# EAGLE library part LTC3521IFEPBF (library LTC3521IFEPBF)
DC/DC Converters Source: Datasheet
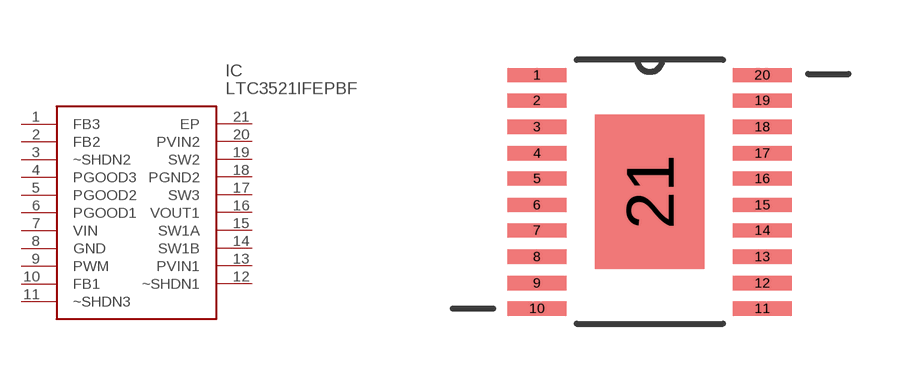
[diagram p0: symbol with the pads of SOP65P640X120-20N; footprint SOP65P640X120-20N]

Designator prefix IC

## LTC3521IFEPBF (Arrow_Part_Number: LTC3521IFEPBF; Description: DC/DC Converters; Height: mm; Manufacturer_Name: Linear Technology; Manufacturer_Part_Number: LTC3521IFEPBF)  [SOP65P640X120-20N]
1  FB3
2  FB2
3  ~SHDN2
4  PGOOD3
5  PGOOD2
6  PGOOD1
7  VIN
8  GND
9  PWM
10  FB1
11  ~SHDN3
12  ~SHDN1
13  PVIN1
14  SW1B
15  SW1A
16  VOUT1
17  SW3
18  PGND2
19  SW2
20  PVIN2
21  EP

## Footprint SOP65P640X120-20N (pad centres in mm)
SOP65P640X120-20N
smd 1.473 x 0.356: 1 -2.819,2.921; 2 -2.819,2.286; 3 -2.819,1.626; 4 -2.819,0.965; 5 -2.819,0.33; 6 -2.819,-0.33; 7 -2.819,-0.965; 8 -2.819,-1.626; 9 -2.819,-2.286; 10 -2.819,-2.921; 11 2.819,-2.921; 12 2.819,-2.286; 13 2.819,-1.626; 14 2.819,-0.965; 15 2.819,-0.33; 16 2.819,0.33; 17 2.819,0.965; 18 2.819,1.626; 19 2.819,2.286; 20 2.819,2.921
smd 2.743 x 3.861: 21 0,0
